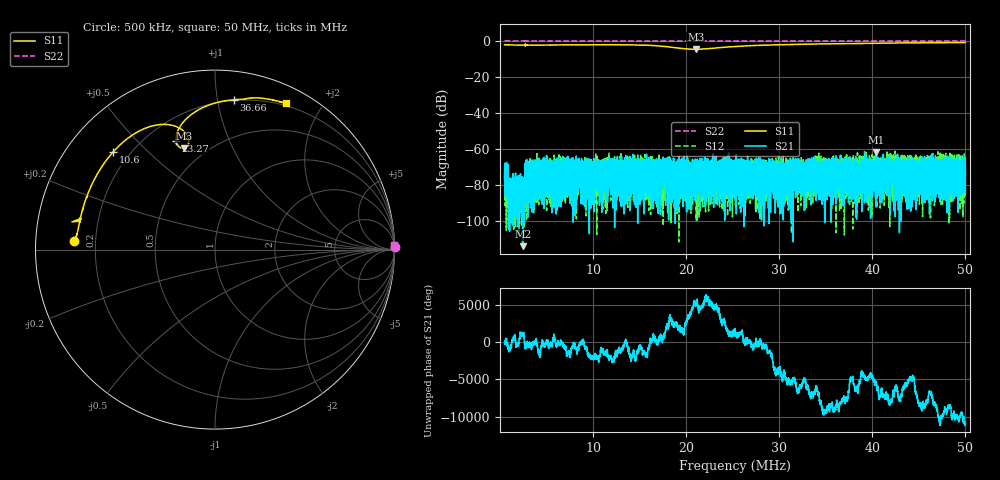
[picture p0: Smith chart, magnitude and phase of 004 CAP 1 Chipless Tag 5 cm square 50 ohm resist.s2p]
!  26/06/2025  15:17:39
! Ref Plane: 0.000 mm
# MHZ S MA R  50
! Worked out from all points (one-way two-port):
!   10001 points, 500 kHz to 50 MHz, reference 50 ohm
!   highest |S21| = -61.66 dB at 40.44 MHz (marker M1); lowest = -113.7 dB at 2.47 MHz (marker M2)
!   lowest |S11| = -4.6 dB at 21.04 MHz (marker M3), VSWR 3.87, Z = 19.3 + j33.3 ohm
!   |S11| at or under -10 dB: nowhere
!   |S22| runs from -0.3 to 0.3 dB; largest |S21 - S12| = 0.0014
!   S11 on the Smith chart (normalised r, x): 500 kHz: 0.12, +0.03; 10.6 MHz: 0.14, +0.39; 23.27 MHz: 0.32, +0.66; 36.66 MHz: 0.20, +1.12; 50 MHz: 0.17, +1.58
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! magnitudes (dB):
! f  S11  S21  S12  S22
! 500 kHz  -2.1  -72.7  -73.5  0.0
! 1.134 MHz  -2.2  -81.6  -94.2  0.0
! 2.47 MHz  -2.3  -113.7  -81.3  0.0
! 2.96 MHz  -2.3  -78.4  -71.4  0.0
! 3.188 MHz  -2.3  -73.9  -74.9  0.0
! 8.752 MHz  -2.1  -77.0  -80.3  0.0
! 10.6 MHz  -2.1  -65.9  -67.0  0.0
! 17 MHz  -2.7  -95.7  -78.1  0.0
! 21.04 MHz  -4.6  -72.8  -77.3  0.0
! 23.27 MHz  -3.8  -77.1  -77.4  0.0
! 25.25 MHz  -3.1  -83.1  -74.2  0.0
! 27.52 MHz  -2.5  -75.0  -73.3  0.0
! 33.5 MHz  -1.7  -75.9  -66.6  0.0
! 36.66 MHz  -1.5  -87.3  -68.4  0.0
! 38.4 MHz  -1.4  -71.2  -73.8  0.0
! 38.93 MHz  -1.4  -69.9  -75.5  0.0
! 40.44 MHz  -1.3  -61.7  -63.6  0.0
! 41.75 MHz  -1.2  -77.4  -68.3  0.0
! 46.04 MHz  -1.0  -75.5  -67.3  0.0
! 47.28 MHz  -0.9  -89.1  -72.9  0.0
! 49.72 MHz  -0.8  -74.3  -79.9  0.0
! 50 MHz  -0.8  -83.4  -74.8  0.0
